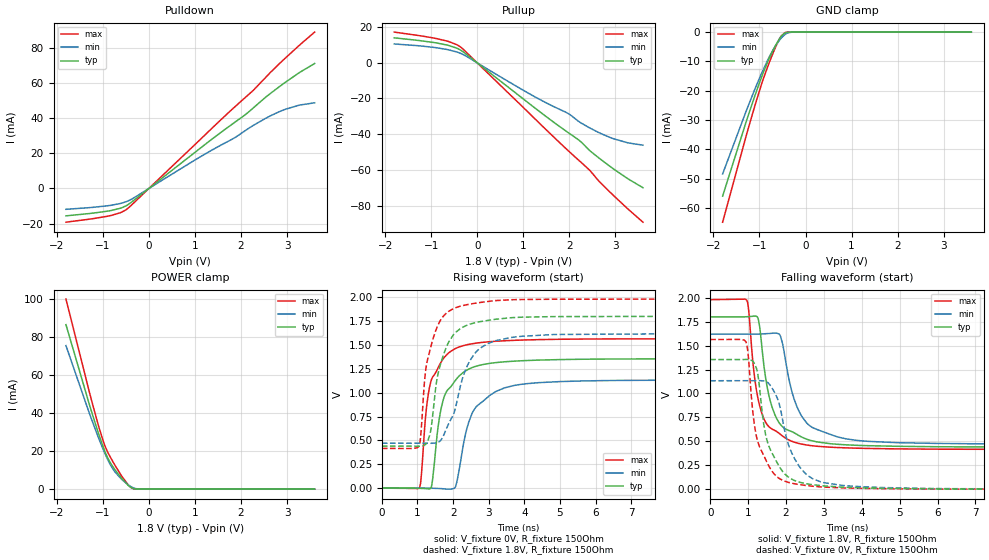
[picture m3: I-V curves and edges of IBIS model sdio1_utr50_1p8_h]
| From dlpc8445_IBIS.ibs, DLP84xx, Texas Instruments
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|   utr50_1p8_h
[Model]   sdio1_utr50_1p8_h
Model_type   I/O
Polarity   Non-Inverting
Enable   Active-High
Vinl = 0
Vinh = 0.8
Vmeas = 0.9
Vref = 1.8
Cref = 2pF
Rref = 100000
|   typ   min   max
C_comp   4.352pF   3.998pF   4.608pF
[Voltage Range]   1.8   1.62   1.98
[Temperature Range]   27   150   -40
[Pullup Reference]   1.8   1.62   1.98
[Pulldown Reference]   0   0   0
[Power Clamp Reference]   1.8   1.62   1.98
[GND Clamp Reference]   0   0   0
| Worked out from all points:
|   slope of the pulldown table from 0 to 0.27 V, typ, clamps not added: 48.4 ohm
|   slope of the pullup table from 0 to 0.27 V, typ, clamps not added: 49.2 ohm
|   GND clamp passes 1 mA (typ) near -0.50 V on its own axis
|   POWER clamp passes 1 mA (typ) near -0.39 V on its own axis
|   falling waveform, V_fixture 1.8V, R_fixture 150Ohm: 20-80 % time 439ps typ, 561ps min, 368ps max; typ from 1.8 V to 0.44 V
|   rising waveform, V_fixture 0V, R_fixture 150Ohm: 20-80 % time 501ps typ, 639ps min, 422ps max; typ from 0 V to 1.35 V
|   rising waveform, V_fixture 1.8V, R_fixture 150Ohm: 20-80 % time 462ps typ, 658ps min, 404ps max; typ from 0.44 V to 1.8 V
|   falling waveform, V_fixture 0V, R_fixture 150Ohm: 20-80 % time 478ps typ, 562ps min, 426ps max; typ from 1.35 V to 0 V
[Pulldown]
|   Voltage   I(typ)   I(min)   I(max)
-1.8V     -15.62mA   -11.89mA   -19.24mA
-892.8mV  -12.91mA   -9.856mA   -15.8mA
-622.8mV  -11.31mA   -8.589mA   -13.88mA
-498.6mV  -9.955mA   -7.593mA   -12.21mA
-298.8mV  -6.192mA   -4.907mA   -7.512mA
1.364V    28.05mA    21.85mA    34.25mA
1.861V    37.71mA    28.94mA    46.48mA
2.12V     42.7mA     33.52mA    52.58mA
2.531V    52.01mA    39.99mA    63.25mA
2.974V    60.82mA    45.32mA    74.7mA
3.26V     65.99mA    47.5mA     81.57mA
3.6V      71.36mA    48.92mA    89.3mA
[GND Clamp]
|   Voltage   I(typ)   I(min)   I(max)
-1.8V     -55.9mA    -48.35mA   -64.79mA
-1.287V   -30.48mA   -26.87mA   -35.27mA
-1.109V   -22.12mA   -19.8mA    -25.59mA
-946.8mV  -15.01mA   -13.77mA   -17.35mA
-790.2mV  -8.997mA   -8.533mA   -10.48mA
-622.8mV  -3.762mA   -4.011mA   -4.148mA
-541.8mV  -1.721mA   -2.298mA   -1.693mA
-450mV    -363uA     -857.5uA   -221.8uA
-347.4mV  -20.25uA   -138.5uA   -4.046uA
-234mV    -328.5nA   -10.21uA   -105.1nA
3.6V      0A         0A         0A
[Pullup]
|   Voltage   I(typ)   I(min)   I(max)
-1.8V     14.01mA    10.58mA    17.23mA
-887.4mV  11.16mA    8.467mA    13.62mA
-628.2mV  9.803mA    7.341mA    12.01mA
-363.6mV  7.163mA    5.33mA     8.904mA
1.213V    -24.52mA   -18.49mA   -30.38mA
1.969V    -39mA      -28.31mA   -49.09mA
2.201V    -43.2mA    -32.8mA    -54.54mA
2.439V    -49.08mA   -36.44mA   -60.13mA
2.639V    -53.27mA   -39.09mA   -66.23mA
2.963V    -59.54mA   -42.57mA   -74.45mA
3.249V    -64.59mA   -44.7mA    -81.37mA
3.6V      -70.03mA   -46.18mA   -89.35mA
[POWER Clamp]
|   Voltage   I(typ)   I(min)   I(max)
-1.8V     86.44mA    75.43mA    99.9mA
-1.287V   44.12mA    39.56mA    50.59mA
-1.109V   30.39mA    27.98mA    34.62mA
-984.6mV  21.72mA    20.51mA    24.79mA
-898.2mV  16.68mA    15.82mA    19.69mA
-741.6mV  10.42mA    9.224mA    12.8mA
-595.8mV  5.776mA    5.267mA    7.057mA
-450mV    2.018mA    2.285mA    2.308mA
-390.6mV  933.1uA    1.359mA    950.1uA
-320.4mV  226.2uA    591.6uA    146.8uA
-147.6mV  917.8nA    14.06uA    197.8nA
3.6V      0A         0A         0A
[Ramp]
R_load = 150
|   typ   min   max
dV/dt_r   0.812415/5.03508e-10   0.67926/6.40769e-10   0.937939/4.22202e-10
dV/dt_f   0.81606/4.37099e-10   0.689308/5.58509e-10   0.938433/3.67441e-10
[Falling Waveform]
V_fixture = 1.8V
V_fixture_min = 1.62V
V_fixture_max = 1.98V
R_fixture = 150Ohm
C_fixture = 0F
|   Time   V(typ)   V(min)   V(max)
0s        1.8V       1.619V     1.98V
965ps     1.802V     1.62V      1.976V
1.14ns    1.807V     1.62V      1.275V
1.245ns   1.799V     1.62V      980.8mV
1.59ns    914.9mV    1.627V     639.5mV
1.86ns    672.4mV    1.593V     570.5mV
2.145ns   602.9mV    1.036V     501.8mV
2.595ns   515.7mV    673.5mV    458.9mV
3.61ns    463mV      524mV      431.3mV
10ns      439.7mV    470.6mV    415.8mV
[Rising Waveform]
V_fixture = 0V
V_fixture_min = 0V
V_fixture_max = 0V
R_fixture = 150Ohm
C_fixture = 0F
|   Time   V(typ)   V(min)   V(max)
0s        324.9uV    852.1uV    192.1uV
1.06ns    -1.973mV   598uV      4.757mV
1.245ns   -4.794mV   582.9uV    814.9mV
1.375ns   -806.9uV   -698.8uV   1.116V
1.675ns   852.7mV    -5.065mV   1.328V
2.105ns   1.147V     64.83mV    1.469V
2.355ns   1.229V     577.3mV    1.499V
2.56ns    1.266V     804mV      1.514V
3.445ns   1.323V     1.05V      1.543V
10ns      1.354V     1.133V     1.563V
[Rising Waveform]
V_fixture = 1.8V
V_fixture_min = 1.62V
V_fixture_max = 1.98V
R_fixture = 150Ohm
C_fixture = 0F
|   Time   V(typ)   V(min)   V(max)
0s        439.7mV    470.6mV    415.8mV
1.04ns    439.1mV    470.3mV    436.4mV
1.095ns   440.4mV    470.3mV    567.2mV
1.225ns   457.4mV    470.3mV    1.219V
1.375ns   610.6mV    470mV      1.481V
1.575ns   1.194V     480.1mV    1.707V
2.035ns   1.617V     798.3mV    1.884V
2.475ns   1.717V     1.337V     1.927V
3.185ns   1.768V     1.543V     1.964V
10ns      1.8V       1.619V     1.98V
[Falling Waveform]
|Gnd
V_fixture = 0V
V_fixture_min = 0V
V_fixture_max = 0V
R_fixture = 150Ohm
C_fixture = 0F
|   Time   V(typ)   V(min)   V(max)
0s        1.354V     1.133V     1.563V
940ps     1.355V     1.133V     1.541V
1.005ns   1.354V     1.133V     1.394V
1.135ns   1.332V     1.133V     772.4mV
1.245ns   1.225V     1.134V     512.7mV
1.505ns   501.4mV    1.117V     275.4mV
1.935ns   173.9mV    673.9mV    88.56mV
2.31ns    78.28mV    263.1mV    51.06mV
2.98ns    34.88mV    69.47mV    22.43mV
10ns      324.9uV    858.2uV    192uV
